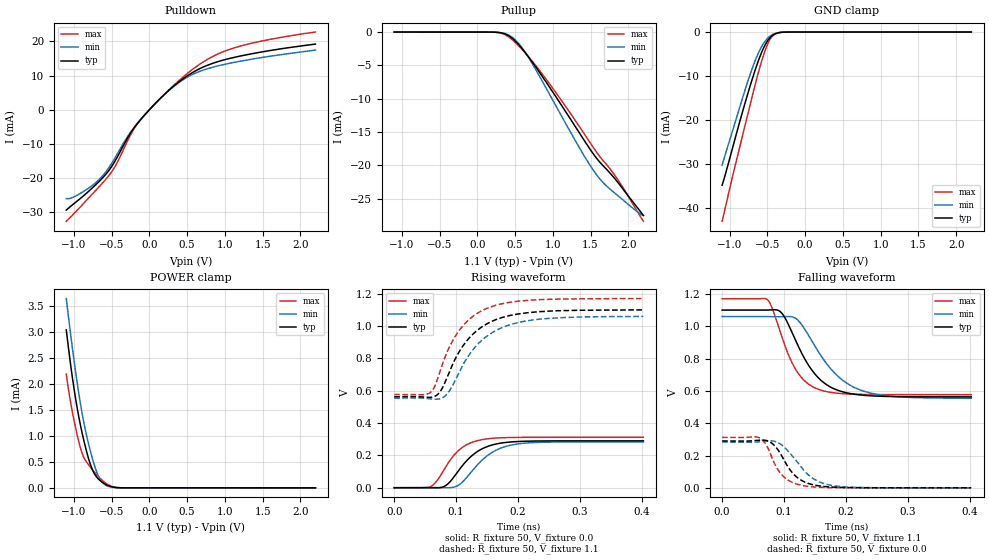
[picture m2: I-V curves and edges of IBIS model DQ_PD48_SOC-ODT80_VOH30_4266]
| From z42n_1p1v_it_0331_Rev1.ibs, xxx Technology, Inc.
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| DQ_PD48_SOC-ODT80_VOH30_4266
| (48 Ohm Pulldown, 80 Ohm System ODT Setting, VOH=VDDQ/3.0, 3200-4266Mbps)
[Model]   DQ_PD48_SOC-ODT80_VOH30_4266
Model_type   I/O
Vinl = 123.333mV
Vinh = 243.333mV
Vmeas = 183.333mV
Vref = 0.0mV
Cref = 0.0pF
Rref = 80.000Ohm
|   typ   min   max
|C_comp   0.834pF   0.784pF   0.884pF
C_comp_pullup   0.4170pF   0.3920pF   0.4420pF
C_comp_pulldown   0.4170pF   0.3920pF   0.4420pF
| Note: C_comp changes when the ODT circuit is enabled.
[Model Spec]
| Input threshold voltage corners
Vinl   0.1233V   0.1167V   0.1350V
Vinh   0.2433V   0.2367V   0.2550V
| Measurement voltage corners
Vmeas   0.1833V   0.1767V   0.1950V
| Timing spec test load voltage corners
Vref   0.0000V   0.0000V   0.0000V
| Dynamic Overshoot Parameters from LPDDR4 Specification
D_overshoot_ampl_h   0.30   NA   NA
D_overshoot_ampl_l   0.30   NA   NA
D_overshoot_area_h   0.1n   NA   NA
D_overshoot_area_l   0.1n   NA   NA
[Voltage Range]   1.1000V   1.0600V   1.1700V
[Pullup Reference]   1.1000V   1.0600V   1.1700V
| Junction Temperature (Ambient temp is 35C typ 95C min -40C max)
[Temperature Range]   50.0   110.0   -40.0
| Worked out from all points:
|   slope of the pulldown table from 0 to 0.165 V, typ, clamps not added: 43.9 ohm
|   slope of the pullup table from 0 to 0.165 V, typ, clamps not added: 26 kohm
|   GND clamp passes 1 mA (typ) near -0.45 V on its own axis
|   POWER clamp passes 1 mA (typ) near -0.88 V on its own axis
|   rising waveform, R_fixture 50, V_fixture 0.0: 20-80 % time 43ps typ, 46ps min, 37.6ps max; typ from 0 V to 0.29 V
|   falling waveform, R_fixture 50, V_fixture 1.1: 20-80 % time 48.9ps typ, 61.1ps min, 38.9ps max; typ from 1.1 V to 0.563 V
|   rising waveform, R_fixture 50, V_fixture 1.1: 20-80 % time 56.5ps typ, 60.5ps min, 52.2ps max; typ from 0.563 V to 1.1 V
|   falling waveform, R_fixture 50, V_fixture 0.0: 20-80 % time 32.5ps typ, 40.5ps min, 27.8ps max; typ from 0.29 V to 0 V
[Pulldown]
|   Voltage   I(typ)   I(min)   I(max)
-1.1V     -29.31mA   -25.95mA   -32.57mA
-918.5mV  -26mA      -24.49mA   -28.5mA
-661.1mV  -20.85mA   -20.29mA   -22.4mA
-466.4mV  -15.43mA   -14.48mA   -17.04mA
-245.3mV  -6.697mA   -6.46mA    -7.234mA
-123.2mV  -3.076mA   -3.063mA   -3.08mA
239.8mV   5.304mA    5.231mA    5.394mA
563.2mV   10.75mA    10.22mA    11.64mA
847mV     13.62mA    12.47mA    15.65mA
1.157V    15.46mA    13.99mA    18.29mA
1.636V    17.43mA    15.76mA    20.71mA
2.2V      19.18mA    17.44mA    22.7mA
[GND Clamp]
|   Voltage   I(typ)   I(min)   I(max)
-1.1V     -34.74mA   -30.21mA   -42.91mA
-941.6mV  -25.02mA   -21.26mA   -31.32mA
-796.4mV  -16.11mA   -13.14mA   -21.19mA
-723.8mV  -11.93mA   -9.349mA   -16.1mA
-664.4mV  -8.736mA   -6.578mA   -12.07mA
-588.5mV  -5.112mA   -3.681mA   -7.298mA
-519.2mV  -2.565mA   -1.832mA   -3.66mA
-466.4mV  -1.295mA   -941.3uA   -1.69mA
-413.6mV  -565uA     -416.7uA   -620.3uA
-357.5mV  -191.8uA   -144.1uA   -173.1uA
-258.5mV  -16.05uA   -14.26uA   -9.823uA
2.2V      0A         0A         0A
[Pullup]
|   Voltage   I(typ)   I(min)   I(max)
-1.1V     3.138uA    4.837uA    1.415uA
229.9mV   -22.54uA   -23.04uA   -23.32uA
342.1mV   -191.9uA   -157uA     -262.8uA
434.5mV   -694.3uA   -568.3uA   -877.6uA
553.3mV   -1.948mA   -1.797mA   -2.113mA
688.6mV   -3.877mA   -3.992mA   -3.837mA
1.065V    -10.1mA    -11.55mA   -9.452mA
1.375V    -15.52mA   -17.78mA   -14.56mA
1.576V    -18.87mA   -21.34mA   -17.96mA
1.685V    -20.27mA   -22.79mA   -19.52mA
1.857V    -22.47mA   -24.49mA   -22.07mA
2.2V      -27.52mA   -27.51mA   -28.38mA
[POWER Clamp]
|   Voltage   I(typ)   I(min)   I(max)
-1.1V     3.033mA    3.633mA    2.184mA
-1.041V   2.345mA    2.929mA    1.625mA
-981.2mV  1.753mA    2.275mA    1.183mA
-911.9mV  1.2mA      1.611mA    764.4uA
-852.5mV  818.4uA    1.149mA    543.6uA
-779.9mV  447.9uA    701.6uA    396.3uA
-713.9mV  239.3uA    373uA      278.6uA
-657.8mV  146.8uA    178.8uA    190.7uA
-598.4mV  83.67uA    71.98uA    113uA
-496.1mV  20.08uA    12.31uA    25.7uA
-380.6mV  1.605uA    1.128uA    1.335uA
2.2V      0A         0A         0A
[Ramp]
|   typ   min   max
| 20% - 80%
dV/dt_r   173.93m/42.98p   169.87m/46.04p   187.31m/37.61p
dV/dt_f   322.28m/48.94p   303.39m/61.11p   355.99m/38.85p
| 25% - 75%
|dV/dt_r   144.94m/34.27p   141.56m/36.75p   156.10m/29.83p
|dV/dt_f   268.57m/39.08p   252.83m/48.77p   296.66m/30.94p
R_load = 50
[Rising Waveform]
R_fixture = 50
V_fixture = 0.0
|   Time   V(typ)   V(min)   V(max)
0s        301.2uV    248.7uV    223.8uV
58ps      213.5uV    308.8uV    5.501mV
68ps      172.9uV    -225.2uV   39.05mV
80ps      7.078mV    -404.7uV   109.8mV
105ps     112mV      19.18mV    234.5mV
123ps     190.6mV    91.34mV    277.2mV
140ps     237.3mV    164.6mV    296.5mV
167ps     272.8mV    237.4mV    308.1mV
204ps     286.9mV    273.5mV    311.7mV
402ps     290.2mV    283.4mV    312.4mV
[Falling Waveform]
R_fixture   = 50
V_fixture   = 1.1
V_fixture_min = 1.06
V_fixture_max = 1.17
|   Time   V(typ)   V(min)   V(max)
0s        1.1V       1.06V      1.17V
73ps      1.1V       1.06V      1.164V
81ps      1.101V     1.059V     1.11V
94ps      1.09V      1.059V     962.6mV
117ps     925.3mV    1.052V     743.8mV
134ps     793.2mV    977.8mV    658.9mV
155ps     681.9mV    844.4mV    610.2mV
191ps     598.2mV    676.6mV    583.8mV
231ps     571.9mV    595.1mV    578mV
402ps     562.9mV    554.3mV    576.7mV
[Rising Waveform]
R_fixture   = 50
V_fixture   = 1.1
V_fixture_min = 1.06
V_fixture_max = 1.17
|   Time   V(typ)   V(min)   V(max)
0s        562.7mV    553.9mV    576.6mV
58ps      559.3mV    549.8mV    588.4mV
67ps      568.5mV    547.4mV    641.5mV
80ps      634.8mV    561.4mV    788.2mV
95ps      770mV      638mV      914.4mV
113ps     888.5mV    774.4mV    1.011V
132ps     967.7mV    876.3mV    1.074V
155ps     1.025V     952.2mV    1.118V
227ps     1.087V     1.04V      1.162V
402ps     1.1V       1.06V      1.17V
[Falling Waveform]
R_fixture = 50
V_fixture = 0.0
|   Time   V(typ)   V(min)   V(max)
0s        290.3mV    283.5mV    312.5mV
58ps      294.4mV    284.6mV    312.5mV
76ps      286.6mV    291.5mV    228.6mV
86ps      255.2mV    286.9mV    139.2mV
97ps      192.6mV    262.9mV    78.1mV
112ps     99.68mV    203.3mV    36.01mV
129ps     44.27mV    121.7mV    15.18mV
153ps     14.35mV    43.87mV    4.659mV
186ps     3.401mV    10.3mV     1.097mV
402ps     370.7uV    348.6uV    245.1uV
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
